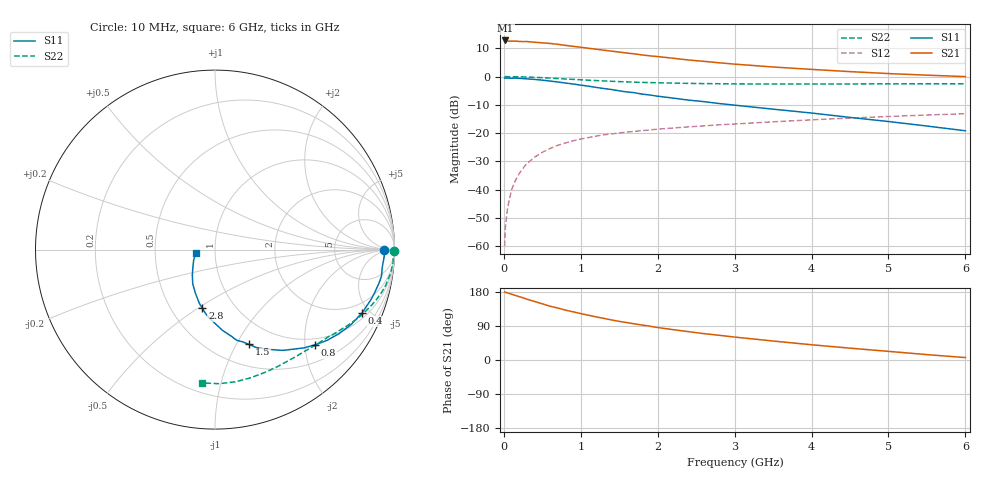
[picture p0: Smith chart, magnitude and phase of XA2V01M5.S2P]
! SIEMENS Discrete & RF Semiconductors
! BFY180
! Si NPN RF Bipolar Junction Transistor in MICRO-X
! VCE = 2 V  IC = 1.5 mA
! Common Emitter S-Parameters:  May  1997
# GHz  S  MA  R  50
!  f  S11  S21  S12  S22
! GHz  MAG  ANG  MAG  ANG  MAG  ANG  MAG  ANG
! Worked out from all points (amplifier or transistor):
!   36 points, 10 MHz to 6 GHz, reference 50 ohm
!   highest |S21| = 12.8 dB at 20 MHz (marker M1)
!   |S21| within 3 dB of that: start of sweep to 1.173 GHz
!   unconditionally stable (mu >= 1): 2.932 GHz to end of sweep
!   at 250 MHz: K = 0.10, MSG = 22.4 dB, |S12| = -32.4 dB
!   at 1.4 GHz: K = 0.63, MSG = 14.6 dB, |S12| = -20.3 dB
!   at 6 GHz: K = 1.08, MAG = 4.8 dB, |S12| = -13.1 dB
!   S11 on the Smith chart (normalised r, x): 10 MHz: 34, -3; 400 MHz: 1.30, -4.49; 800 MHz: 0.85, -2.22; 1.5 GHz: 0.73, -1.13; 2.8 GHz: 0.71, -0.52; 6 GHz: 0.80, -0.03
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0.01  0.9425 -0.3  4.234 179.5  0.001 91.0  0.9961 -0.3
0.02  0.9455 -1.4  4.362 178.6  0.0022 85.7  0.9999 -0.7
0.05  0.9422 -2.9  4.235 177.0  0.0049 85.6  0.9958 -1.6
0.1  0.9371 -6.0  4.243 173.7  0.0099 86.6  0.9938 -3.1
0.15  0.9393 -9.2  4.249 170.4  0.0145 85.0  0.9944 -4.7
0.3  0.9131 -17.7  4.172 160.5  0.0289 78.5  0.9804 -9.2
0.4  0.8919 -23.3  4.052 154.4  0.0376 75.2  0.9711 -12.0
0.6  0.8349 -34.1  3.864 141.9  0.0534 68.1  0.9411 -17.3
0.8  0.7697 -43.6  3.572 131.6  0.0669 62.5  0.9079 -22.0
1  0.7068 -51.7  3.309 122.5  0.0787 57.3  0.8791 -26.2
1.1  0.6766 -56.1  3.168 118.1  0.0835 55.1  0.8636 -28.0
1.2  0.6448 -59.9  3.059 113.7  0.0886 53.2  0.8512 -29.8
1.5  0.5604 -70.3  2.719 101.9  0.1006 48.5  0.8161 -34.7
1.7  0.5189 -76.6  2.522 95.3  0.1074 45.9  0.796 -37.6
2  0.4504 -84.9  2.261 85.6  0.1177 42.9  0.7783 -41.9
2.2  0.4166 -89.2  2.114 80.1  0.1233 40.7  0.7673 -44.7
2.6  0.361 -98.3  1.863 69.6  0.1343 37.6  0.7524 -49.8
2.8  0.334 -102.2  1.755 65.2  0.1404 36.1  0.7483 -52.3
3.5  0.2655 -114.4  1.48 50.1  0.1586 31.2  0.7392 -61.2
4.5  0.1898 -131.7  1.225 31.2  0.1848 23.9  0.7411 -74.3
5.5  0.1336 -153.0  1.061 14.2  0.2091 16.3  0.7474 -88.3
6  0.11 -170.6  1 6.4  0.2204 12.0  0.7465 -95.4
